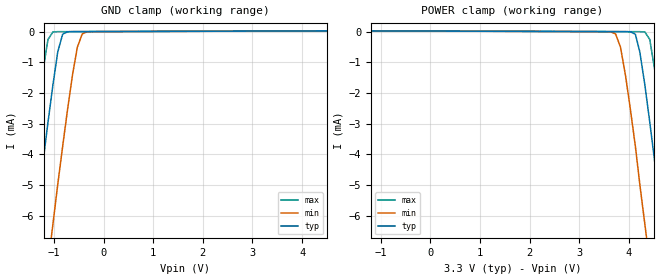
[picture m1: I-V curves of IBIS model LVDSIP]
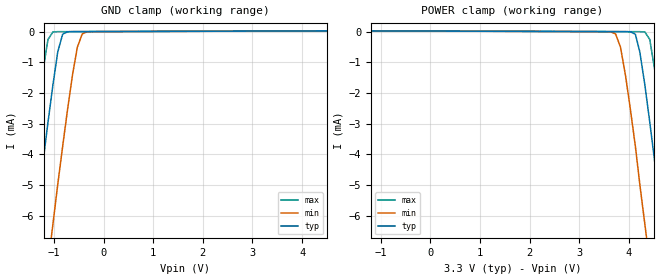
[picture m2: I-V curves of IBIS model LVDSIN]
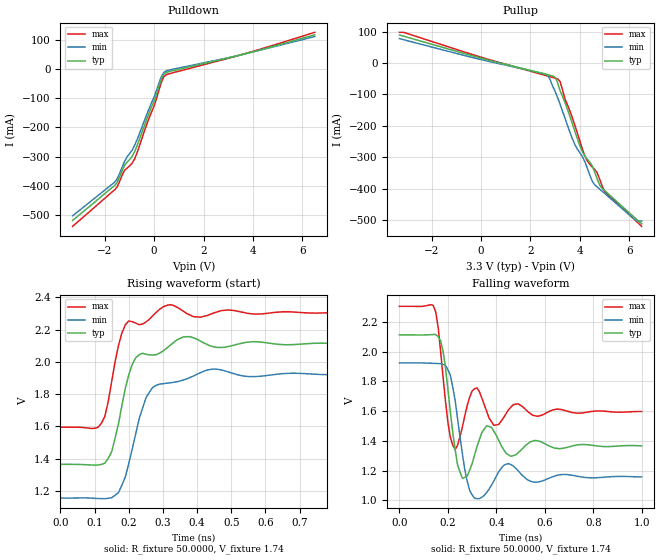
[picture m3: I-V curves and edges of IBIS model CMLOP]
|   National Semiconductor Corporation
|   IBIS Model of DS32ELX0124
[IBIS Ver]   4.0
[File name]   ds32elx0421.ibs
[File Rev]   1.0
[Notes]
 Created By  Pegah Alavi, Shrikant Kadadevar
   Revision History
   1.0   | Initial Release
[Date]   05/20/2009
[Source]  Generated by National Semincoductor Corporation.
[Disclaimer]
(C) Copyright National Semiconductor Corporation 2009
   All rights reserved
National Semiconductor Corporation hereby grants the
user of this IBIS model a non-exclusive, nontransferable
license to use this IBIS model under the following terms.
Before using this IBIS model, the user should read this
license.  If the user does not accept these terms,  the
IBIS model should be returned to National within 30 days.
The user is granted this license only to use the
IBIS model and is not granted rights to sell, load, rent,
lease or license the IBIS model in whole or in part, or in
modified form to anyone other than user. User may modify
the IBIS model to suit its specific applications but rights
to derivative works and such modifications shall belong to
National.
This IBIS model is provided on an "AS IS" basis and
National makes absolutely no warranty with respect to the
information contained herein.NATIONAL DISCLAIMS AND CUSTOMER
WAIVES ALL WARRANTIES, EXPRESS OR IMPLIED, INCLUDING
WARRANTIES OF MERCHANTABILITY OR FITNESS FOR A PARTICULAR
PURPOSE. The entire risk as to quality and performance is
with the Customer. ACCORDINGLY, IN NO EVENT SHALL THE
COMPANY BE LIABLE FOR ANY DAMAGES, WHETHER IN CONTRACT OR
TORT,INCLUDING ANY LOST PROFITS OR OTHER INCIDENTAL,
CONSEQUENTIAL, EXEMPLARY, OR PUNITIVE DAMAGES ARISING OUT
OF THE USE OR APPLICATION OF THE IBIS model provided in
this package.Further, National reserves the right to make
changes without notice to any product herein to improve
reliability, function, or design. National does not convey
any license under patent rights or any other intellectual
property rights, including those of third parties.
National is not obligated to provide maintenance or support
for the licensed IBIS model.
[Copyright]  Copyright 2009, National Semiconductor, All Rights Reserved
[Component]  DS32ELX0421
[Manufacturer]  National Semiconductor Corp
[Package]
|   typ   min   max
R_pkg   0   0   0
L_pkg   0   0   0
C_pkg   0   0   0
[Pin]   signal_name   model_name   R_pin   L_pin   C_pin
1   VDD33_0   POWER
2   NCO   NC
3   GPIO0   CMOSIO
4   GPIO1   CMOSIO
5   DC_B   CMOSI
6   RS   CMOSI
7   VDD25_0   POWER
8   NC1   NC
9   DE_EMPH0   CMOSI
10   DE_EMPH1   CMOSI
11   GPIO2   CMOSI
12   TXOUT1_EN   CMOSI
13   NC2   NC
14   VOD_CTRL   NC
15   VDD25_1   POWER
16   TXOUT0+   CMLOP
17   TXOUT0-   CMLON
18   VDD25_2   POWER
19   TXOUT1+   CMLOP
20   TXOUT1-   CMLON
21   NC3   NC
22   NC4   NC
23   NC5   NC
24   NC6   NC
25   VDD25_3   POWER
26   LF_REF   NC
27   LF_CP   NC
28   VDDPLL   POWER
29   RSVD   CMOSI
30   RESET   CMOSI
31   LOCK   CMOSO
32   SDA   SMBUS
33   SCK   SMBUS
34   SMB_CS   CMOSI
35   VDD25_4   POWER
36   VDD33_1   POWER
37   TXCLKIN+   LVDSIP
38   TXCLKIN-   LVDSIN
39   TXIN0+   LVDSIP
40   TXIN0-   LVDSIN
41   TXIN1+   LVDSIP
42   TXIN1-   LVDSIN
43   TXIN2+   LVDSIP
44   TXIN2-   LVDSIN
45   TXIN3+   LVDSIP
46   TXIN3-   LVDSIN
47   TXIN4+   LVDSIP
48   TXIN4-   LVDSIN
49   DAP   GND
[Diff pin]  inv_pin  vdiff  tdelay_typ  tdelay_min  tdelay_max
16   17   0.0   0.0s   0.0s   0.0s
19   20   0.0   0.0s   0.0s   0.0s
37   38   300m   0.0s   0.0s   0.0s
39   40   300m   0.0s   0.0s   0.0s
41   42   300m   0.0s   0.0s   0.0s
43   44   300m   0.0s   0.0s   0.0s
45   46   300m   0.0s   0.0s   0.0s
47   48   300m   0.0s   0.0s   0.0s
[Package Model] 48 LLP for DS32ELX0421SQ
|   Package Model
[Define Package Model]  48 LLP for DS32ELX0421SQ
[Manufacturer]  National Semiconductor
[OEM] NA
[Description]  Package Model for DS32ELX0421SQ
[Number Of Pins]  49
[Pin Numbers]
49   | 49 = DAP
1   | 1 = L1
2   | 2 = L2
3   | 3 = L3
4   | 4 = L4
5   | 5 = L5
6   | 6 = L6
7   | 7 = L7
8   | 8 = L8
9   | 9 = L9
10   | 10 = L10
11   | 11 = L11
12   | 12 = L12
13   | 13 = L13
14   | 14 = L14
15   | 15 = L15
16   | 16 = L16
17   | 17 = L17
18   | 18 = L18
19   | 19 = L19
20   | 20 = L20
21   | 21 = L21
22   | 22 = L22
23   | 23 = L23
24   | 24 = L24
25   | 25 = L25
26   | 26 = L26
27   | 27 = L27
28   | 28 = L28
29   | 29 = L29
30   | 30 = L30
31   | 31 = L31
32   | 32 = L32
33   | 33 = L33
34   | 34 = L34
35   | 35 = L35
36   | 36 = L36
37   | 37 = L37
38   | 38 = L38
39   | 39 = L39
40   | 40 = L40
41   | 41 = L41
42   | 42 = L42
43   | 43 = L43
44   | 44 = L44
45   | 45 = L45
46   | 46 = L46
47   | 47 = L47
48   | 48 = L48
[Model Data]
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[End Model Data]
[End Package Model]
| Models and submodels in the file (8): LVDSIP (Input), LVDSIN (Input), CMLOP (Output), CMLON (Output), CMOSI (Input), CMOSO (Output), CMOSIO (I/O), SMBUS (I/O_open_drain)
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|   Model LVDSIP
[Model]  LVDSIP
Model_type Input
Polarity   Non-Inverting
Vinh = 2
Vinl = 0
C_comp   219.7fF   219.1fF   220.0fF
[Temperature Range]   25.0000   85.0000   -40.0000
[Voltage Range]   3.3000V   3.1350V   3.4650V
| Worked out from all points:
|   GND clamp passes 1 mA (typ) near -0.95 V on its own axis
[Power Clamp]
|Voltage   I(typ)   I(min)   I(max)
|6.60E+00   -3.34E-02   -3.70E-02   -3.16E-02
-3.3V     33.1uA     33.6uA     31.1uA
3.73V     -2.15uA    -74.1uA    -1.21uA
3.83V     -2.65uA    -507uA     -1.67uA
3.93V     -3.23uA    -1.42mA    -2.12uA
4.13V     -87.3uA    -3.74mA    -3.03uA
4.22V     -667uA     -4.98mA    -3.55uA
4.32V     -1.73mA    -6.26mA    -11.2uA
4.42V     -2.95mA    -7.55mA    -258uA
4.62V     -5.57mA    -10.2mA    -2.53mA
4.72V     -6.91mA    -11.5mA    -3.89mA
4.92V     -9.64mA    -14.1mA    -6.71mA
6.5V      -32mA      -35.6mA    -30.2mA
[GND Clamp]
|Voltage   I(typ)   I(min)   I(max)
-3.3V     -33.4mA    -37mA      -31.6mA
-1.62V    -9.64mA    -14.1mA    -6.71mA
-1.42V    -6.91mA    -11.5mA    -3.89mA
-1.32V    -5.57mA    -10.2mA    -2.53mA
-1.12V    -2.95mA    -7.55mA    -258uA
-1.02V    -1.73mA    -6.26mA    -11.2uA
-924mV    -667uA     -4.98mA    -3.55uA
-825mV    -87.3uA    -3.74mA    -3.03uA
-627mV    -3.23uA    -1.42mA    -2.12uA
-528mV    -2.65uA    -507uA     -1.67uA
-429mV    -2.15uA    -74.1uA    -1.21uA
6.5V      32.6uA     33uA       30.6uA
|   Model LVDSIN
[Model]  LVDSIN
Model_type Input
Polarity   Inverting
Vinh = 2
Vinl = 0
C_comp   219.7fF   219.1fF   220.0fF
[Temperature Range]   25.0000   85.0000   -40.0000
[Voltage Range]   3.3000V   3.1350V   3.4650V
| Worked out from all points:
|   GND clamp passes 1 mA (typ) near -0.95 V on its own axis
[Power Clamp]
|Voltage   I(typ)   I(min)   I(max)
|6.60E+00   -3.34E-02   -3.70E-02   -3.16E-02
-3.3V     33.1uA     33.6uA     31.1uA
3.73V     -2.15uA    -74.1uA    -1.21uA
3.83V     -2.65uA    -507uA     -1.67uA
3.93V     -3.23uA    -1.42mA    -2.12uA
4.13V     -87.3uA    -3.74mA    -3.03uA
4.22V     -667uA     -4.98mA    -3.55uA
4.32V     -1.73mA    -6.26mA    -11.2uA
4.42V     -2.95mA    -7.55mA    -258uA
4.62V     -5.57mA    -10.2mA    -2.53mA
4.72V     -6.91mA    -11.5mA    -3.89mA
4.92V     -9.64mA    -14.1mA    -6.71mA
6.5V      -32mA      -35.6mA    -30.2mA
[GND Clamp]
|Voltage   I(typ)   I(min)   I(max)
-3.3V     -33.4mA    -37mA      -31.6mA
-1.62V    -9.64mA    -14.1mA    -6.71mA
-1.42V    -6.91mA    -11.5mA    -3.89mA
-1.32V    -5.57mA    -10.2mA    -2.53mA
-1.12V    -2.95mA    -7.55mA    -258uA
-1.02V    -1.73mA    -6.26mA    -11.2uA
-924mV    -667uA     -4.98mA    -3.55uA
-825mV    -87.3uA    -3.74mA    -3.03uA
-627mV    -3.23uA    -1.42mA    -2.12uA
-528mV    -2.65uA    -507uA     -1.67uA
-429mV    -2.15uA    -74.1uA    -1.21uA
6.5V      32.6uA     33uA       30.6uA
|   Model CMLOP
[Model]  CMLOP
Model_type Output
Polarity   Non-Inverting
Vmeas =  1.792
Rref =   50.0000
Vref =   1.7415
C_comp   1.5000pF   NA   NA
[Temperature Range]   25.0000   85.0000   -40.0000
[Voltage Range]   3.3000V   3.000V   3.46500V
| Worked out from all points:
|   slope of the pulldown table from 0 to 0.495 V, typ, clamps not added: 5.02 ohm
|   slope of the pullup table from 0 to 0.495 V, typ, clamps not added: 49.3 ohm
|   rising waveform, R_fixture 50.0000, V_fixture 1.74: 20-80 % time 48.4ps typ, 56.4ps min, 39.9ps max; typ from 1.36 V to 2.11 V
|   falling waveform, R_fixture 50.0000, V_fixture 1.74: 20-80 % time 32.3ps typ, 41.2ps min, 25.8ps max; typ from 2.11 V to 1.37 V
[Pulldown]
|Voltage   I(typ)   I(min)   I(max)
-3.3V     -520.1mA   -504.3mA   -540.5mA
-1.6V     -400.1mA   -388.8mA   -414.9mA
-1.5V     -390mA     -377.8mA   -405.3mA
-1.2V     -331.2mA   -317.6mA   -348.3mA
-800mV    -285.5mA   -263.6mA   -310.2mA
-200mV    -148.9mA   -134.1mA   -166.4mA
1.971fV   -109mA     -94.64mA   -125.8mA
300mV     -31.75mA   -23.79mA   -42.53mA
400mV     -15.89mA   -9.943mA   -24.55mA
600mV     -7.505mA   -2.208mA   -15.04mA
3.4V      47.88mA    48.18mA    47.62mA
6.5V      119.3mA    113.5mA    128mA
[Pullup]
|Voltage   I(typ)   I(min)   I(max)
-3.3V     89.88mA    78.28mA    98.51mA
2.6V      -35mA      -34.6mA    -39.02mA
3V        -45.2mA    -90.63mA   -47.86mA
3.1V      -62.58mA   -110mA     -50.2mA
3.2V      -88.08mA   -131.3mA   -58.51mA
3.7V      -194mA     -241.7mA   -174.9mA
4.2V      -296.3mA   -314mA     -295.1mA
4.6V      -347mA     -388.2mA   -339mA
4.8V      -388.5mA   -401.7mA   -369.9mA
5V        -406.4mA   -415.4mA   -408.7mA
6.3V      -498.6mA   -503.7mA   -505.9mA
6.5V      -512.6mA   -503.7mA   -520.5mA
[Ramp]
| variable   typ   min   max
dV/dt_r   456.047m/53.64p   444.032m/59.22p   461.990m/48.80p
dV/dt_f   450.06m/35.89p   449.935m/41.09p   462.100m/35.41p
R_load = 50.00
[Rising Waveform]
R_fixture= 50.0000
V_fixture= 1.74
V_fixture_min= 1.54
V_fixture_max= 1.95
|time   V(typ)   V(min)   V(max)
0s        1.364V     1.155V     1.595V
120ps     1.364V     1.152V     1.619V
150ps     1.443V     1.157V     1.878V
170ps     1.618V     1.19V      2.102V
190ps     1.837V     1.287V     2.229V
220ps     2.024V     1.55V      2.241V
250ps     2.048V     1.775V     2.247V
310ps     2.083V     1.867V     2.349V
450ps     2.093V     1.955V     2.304V
1ns       2.113V     1.923V     2.306V
[Falling Waveform]
R_fixture= 50.0000
V_fixture= 1.74
V_fixture_min= 1.54
V_fixture_max= 1.95
|time   V(typ)   V(min)   V(max)
0s        2.113V     1.925V     2.305V
140ps     2.116V     1.922V     2.31V
180ps     2.003V     1.915V     1.832V
210ps     1.601V     1.844V     1.426V
230ps     1.343V     1.673V     1.343V
260ps     1.149V     1.313V     1.495V
310ps     1.304V     1.016V     1.751V
390ps     1.465V     1.132V     1.505V
460ps     1.297V     1.242V     1.627V
1ns       1.367V     1.158V     1.598V
